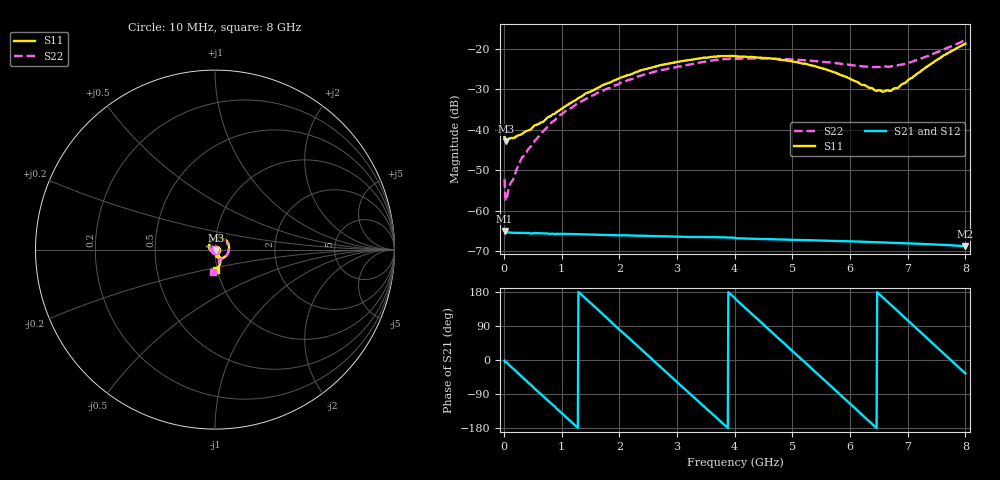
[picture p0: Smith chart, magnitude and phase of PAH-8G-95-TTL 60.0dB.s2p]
! MTS Systemtechnik GmbH
! S-Parameters
! Model: PAH-8G/95-TTL
! Attenuation Step: 60.0dB
! Rohde & Schwarz ZVB8 2Ports - Version 4.11 - 1145.1010k08 SN: 100119
! S2P File Measurements:
! S11 S21 S12 S22
# HZ  S  DB  R  50.00
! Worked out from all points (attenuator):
!   800 points, 10 MHz to 8 GHz, reference 50 ohm
!   highest |S21| = -65.00 dB at 10 MHz (marker M1); lowest = -68.7 dB at 8 GHz (marker M2)
!   lowest |S11| = -42.8 dB at 30 MHz (marker M3), VSWR 1.01, Z = 50.7 - j0.141 ohm
!   |S11| at or under -10 dB: start of sweep to end of sweep
!   |S22| runs from -57.6 to -17.9 dB; largest |S21 - S12| = 1.2e-05
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1e7  -41.80 -16.5  -65.00 -1.6  -64.85 -0.8  -52.24 -62.9
3e7  -42.81 -11.0  -65.39 -6.2  -65.41 -6.4  -57.57 -47.3
6e7  -42.58 -11.4  -65.33 -8.3  -65.34 -8.1  -56.02 -40.3
1.1e8  -42.09 -19.3  -65.41 -16.2  -65.41 -16.2  -53.31 -49.0
2.9e8  -41.20 -47.7  -65.49 -41.5  -65.50 -41.4  -47.46 -84.4
5.6e8  -38.81 -87.0  -65.52 -79.6  -65.55 -79.4  -42.31 -117.0
9.4e8  -35.41 -133.4  -65.69 -132.0  -65.69 -132.0  -36.66 -149.8
1.35e9  -31.74 -172.8  -65.84 171.1  -65.85 171.2  -32.94 -178.6
1.71e9  -29.00 160.1  -65.98 121.0  -66.00 121.5  -30.45 157.5
2.01e9  -27.21 138.7  -66.06 79.1  -66.08 79.4  -28.48 138.3
2.68e9  -24.16 96.8  -66.29 -13.9  -66.28 -13.6  -25.47 100.8
3.44e9  -22.27 53.3  -66.49 -118.3  -66.51 -118.7  -23.29 59.4
4.01e9  -21.88 20.5  -66.79 161.3  -66.80 161.3  -22.49 29.0
4.69e9  -22.48 -16.9  -67.05 67.0  -67.08 66.8  -22.47 -4.9
5.34e9  -24.14 -50.6  -67.30 -23.2  -67.30 -23.2  -22.97 -34.5
5.74e9  -25.87 -67.7  -67.47 -78.8  -67.48 -78.8  -23.54 -49.7
6.44e9  -30.33 -76.1  -67.76 -176.9  -67.82 -176.9  -24.52 -66.2
6.67e9  -30.35 -66.6  -67.88 150.8  -67.91 150.8  -24.46 -67.8
6.84e9  -29.53 -61.2  -67.99 127.1  -68.00 127.1  -24.02 -69.5
7.19e9  -25.93 -56.9  -68.15 77.8  -68.14 78.0  -22.67 -72.7
7.63e9  -21.60 -70.2  -68.44 16.1  -68.46 16.2  -20.13 -82.0
8e9  -18.76 -87.9  -68.75 -35.5  -68.79 -35.4  -17.95 -95.0
